(* Logix 5000 AddOnInstructionDefinition export Banner_RSio_ISD_Device_Information_v1; software revision 33.00 *)

TYPE Banner_RSio_ISD_Data_v1 :   // Tag Data for a Banner ISD Device.
STRUCT
   Safety_Input_Fault : SINT;   // System detected a fault on the safety input. Power cycle required. 1 = True, 0 = False.
   Reserved : SINT;
   Sensor_not_Paired : SINT;   // Si-RF Only. High or Unique sensor that has not been taught (not taught 1, taught 0)
   ISD_Data_Error : SINT;   // 1 = corrupted data was received by the Safety Controller, 0 = data ok.
   Wrong_Actuator : SINT;   // Si-RF sensor detects an actuator with a "received code" that does not match the "expected code" (wrong 1, correct 0).
   Marginal_Range : SINT;   // Si-RF Only. Actuator detected but is staying at the extreme end of detection range (13 to 15 mm away from sensor). 1 = True, 0 = False.
   Actuator_Detected : SINT;   // Si-RF sensor detects an actuator. Note: It does not have to be the taught actuator.
   Output_Error : SINT;   // ISD device detects an output short to voltage or ground. This starts the "switch-off timer" counter. 1= Error detected, 0 = OK.
   Input_1 : SINT;   // ISD device input 1 is on (1) or off (0)
   Input_2 : SINT;   // ISD device input 2 is on (1) or off (0)
   Local_Reset_Expected : SINT;   // An ISD device with latching feature requires a reset. 1 = reset needed. ISD Connect is always 0.
   Operating_Voltage_Warning : SINT;   // Voltage to the ISD device is at limit of specificaitons. 1 = at limit, 0 = OK.
   Operating_Voltage_Error : SINT;   // Voltage to the ISD device is above/over 30 Vdc or below/less 19.2 Vdc limit of range.
   Output_1 : SINT;   // 1 = Output On, 0 = Output Off
   Output_2 : SINT;   // 1 = Output On, 0 = Output Off
   Power_Cycle_Required : SINT;   // 1 = ISD device detects a fault. Power cycled required.
   Fault_Tolerant_Outputs : SINT;   // 1 = ISD device includes 20 minute off delay/fault delay. Always 1 for ISD E-Stop and ISD Connect.
   Local_Reset_Unit : SINT;   // 1 = ISD device includes the latch feature, 0 = device has the auto reset feature. Always 0 for ISD Connect.
   Cascadable : SINT;   // 1 = ISD device includes the cascade feature. Always 1 for ISD E-Stop and ISD Connect.
   High_Coding_Level : SINT;   // Si-RF Only. 1 = Device is High or Unique model, 0 = Low model.
   Teach_ins_Remaining : INT;   // Si-RF Only. Number of teaches remaining for Si-RF devices with high or unique coding.
   Device_Id : INT;   // ISD Device Type 1 = Si-RF. 7 for ISD E-Stop, 9 for ISD Connect.
   Range_Warning_Count : INT;   // Si-RF sensor only. Count of number of range warnings received in the last 60 minutes.
   Output_Switch_Out_Time : INT;   // Delay counter for certain output errors. 0 = inactive, 1 to 20 = remaining minutes to device lockout state. Value = 31 means Timer is Off.
   Number_of_Voltage_Errors : INT;   // 0 to 60 = Number of voltage warnings received in the last 60 seconds.
   Internal_Temperature : REAL;   // Internal temperature of device in Celsius.
   Actuator_Distance : REAL;   // The distance the actuator is from the Si-RF. Value displayed as a percentage of the Si-RF range.
   Supply_Voltage : REAL;   // Actual input voltage detected by the ISD sensor.
   Expected_Company_Name : INT;   // Fixed value of 6.
   Received_Company_Name : INT;   // Si-RF Only. Value received from Sensor. Should match Expected Company Name.
   Expected_Code : INT;   // Si-RF sensor with high or unique coding displays the actuator code taught to the sensor.
   Received_Code : INT;   // Displays actuator code detected by the Si-RF sensor.
   Internal_Error_A : DINT;
   Internal_Error_B : DINT;
END_STRUCT
END_TYPE

TYPE Banner_RSio_ISD_Device_Info_v1 :
STRUCT
   Chain : SINT;   // Enter Chain that will be accessed.
   Device : SINT;   // Enter Device that will be accessed.
   AccessChainDevice : SINT[2];
   RawInfo : SINT[18];
   DeviceInfo : Banner_RSio_ISD_Data_v1;
END_STRUCT
END_TYPE

ADD_ON_INSTRUCTION Banner_RSio_ISD_Device_Information_v1   (* revision 1.0 *)
VAR_IN_OUT
   ISD_Device : Banner_RSio_ISD_Device_Info_v1; {required}
   MSG : MESSAGE; {required}
   Activate : BOOL; {required}
END_VAR
VAR_OUTPUT
   Busy : BOOL; {visible}
   Done : BOOL; {visible}
   Error : BOOL; {visible}
END_VAR
VAR
   Control : DINT; {access None}
   Timer : TIMER := (PRE := 6000); {access None}
   T_Voltage : DINT; {access None}
   T_Temp : DINT; {access None}
   T_Distance : DINT; {access None}
   Temp2 : DINT[31]; {access None}
   Temp1 : DINT[31]; {access None}
   Distance2 : DINT[13] := ([1] := 7, [2] := 8, [3] := 9, [4] := 10, [5] := 11, [6] := 12, [7] := 13, [8] := 14, [9] := 15, [10] := 16, [11] := 17, [12] := 18); {access None}
   Distance1 : DINT[13] := ([0] := 61, [1] := 62, [2] := 65, [3] := 77, [4] := 110, [5] := 133, [6] := 148, [7] := 158, [8] := 163, [9] := 169, [10] := 172, [11] := 176, [12] := 180); {access None}
   IndexD : DINT; {access None}
   IndexT : DINT; {access None}
   Shift_T : DINT; {access None}
END_VAR

ROUTINE Logic   (* ladder *)
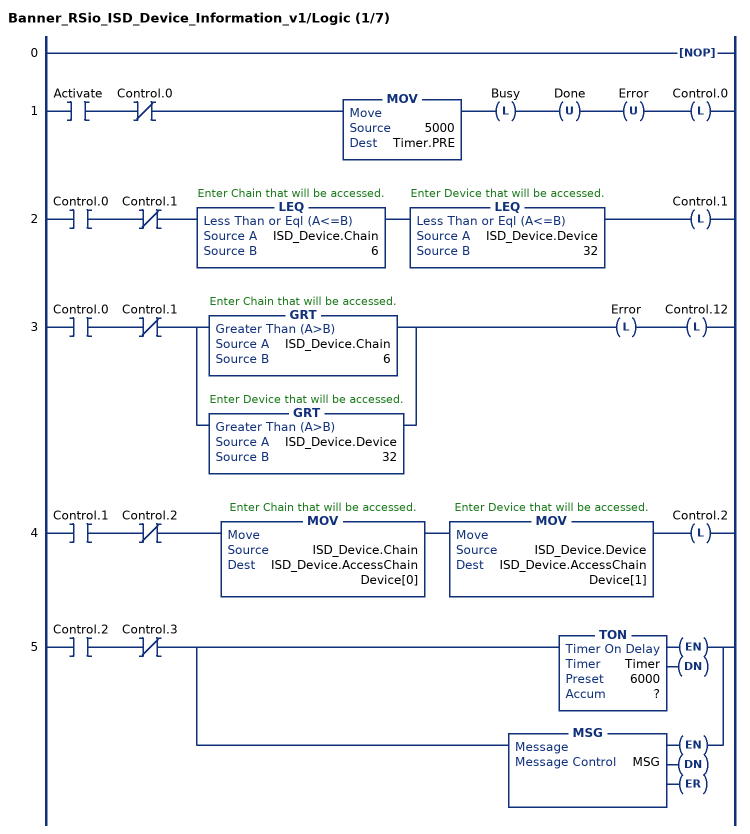
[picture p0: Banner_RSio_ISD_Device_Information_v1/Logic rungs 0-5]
   0: NOP();
   1: XIC(Activate)XIO(Control.0)MOV(5000,Timer.PRE)OTL(Busy)OTU(Done)OTU(Error)OTL(Control.0);
   2: XIC(Control.0)XIO(Control.1)LEQ(ISD_Device.Chain,6)LEQ(ISD_Device.Device,32)OTL(Control.1);
   3: XIC(Control.0)XIO(Control.1)[GRT(ISD_Device.Chain,6) ,GRT(ISD_Device.Device,32) ]OTL(Error)OTL(Control.12);
   4: XIC(Control.1)XIO(Control.2)MOV(ISD_Device.Chain,ISD_Device.AccessChainDevice[0])MOV(ISD_Device.Device,ISD_Device.AccessChainDevice[1])OTL(Control.2);
   5: XIC(Control.2)XIO(Control.3)[TON(Timer,?,?) ,MSG(MSG) ];
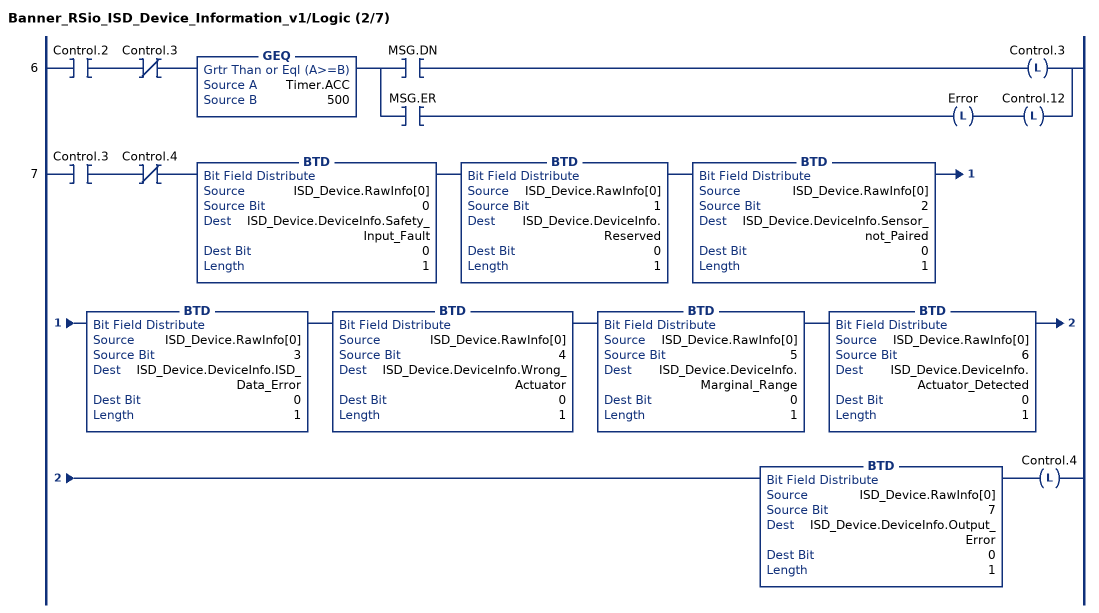
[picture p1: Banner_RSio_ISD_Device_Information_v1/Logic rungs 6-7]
   6: XIC(Control.2)XIO(Control.3)GEQ(Timer.ACC,500)[XIC(MSG.DN) OTL(Control.3) ,XIC(MSG.ER) OTL(Error) OTL(Control.12) ];
   7: XIC(Control.3)XIO(Control.4)BTD(ISD_Device.RawInfo[0],0,ISD_Device.DeviceInfo.Safety_Input_Fault,0,1)BTD(ISD_Device.RawInfo[0],1,ISD_Device.DeviceInfo.Reserved,0,1)BTD(ISD_Device.RawInfo[0],2,ISD_Device.DeviceInfo.Sensor_not_Paired,0,1)BTD(ISD_Device.RawInfo[0],3,ISD_Device.DeviceInfo.ISD_Data_Error,0,1)BTD(ISD_Device.RawInfo[0],4,ISD_Device.DeviceInfo.Wrong_Actuator,0,1)BTD(ISD_Device.RawInfo[0],5,ISD_Device.DeviceInfo.Marginal_Range,0,1)BTD(ISD_Device.RawInfo[0],6,ISD_Device.DeviceInfo.Actuator_Detected,0,1)BTD(ISD_Device.RawInfo[0],7,ISD_Device.DeviceInfo.Output_Error,0,1)OTL(Control.4);
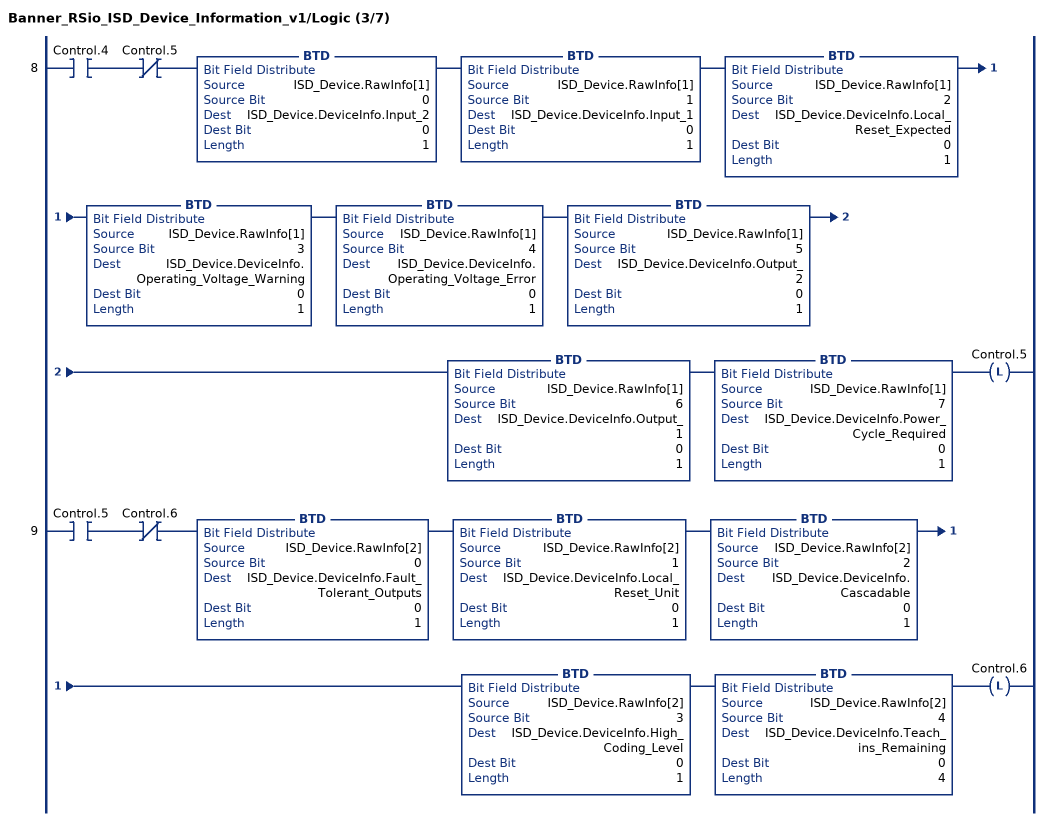
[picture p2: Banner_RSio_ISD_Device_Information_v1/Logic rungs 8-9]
   8: XIC(Control.4)XIO(Control.5)BTD(ISD_Device.RawInfo[1],0,ISD_Device.DeviceInfo.Input_2,0,1)BTD(ISD_Device.RawInfo[1],1,ISD_Device.DeviceInfo.Input_1,0,1)BTD(ISD_Device.RawInfo[1],2,ISD_Device.DeviceInfo.Local_Reset_Expected,0,1)BTD(ISD_Device.RawInfo[1],3,ISD_Device.DeviceInfo.Operating_Voltage_Warning,0,1)BTD(ISD_Device.RawInfo[1],4,ISD_Device.DeviceInfo.Operating_Voltage_Error,0,1)BTD(ISD_Device.RawInfo[1],5,ISD_Device.DeviceInfo.Output_2,0,1)BTD(ISD_Device.RawInfo[1],6,ISD_Device.DeviceInfo.Output_1,0,1)BTD(ISD_Device.RawInfo[1],7,ISD_Device.DeviceInfo.Power_Cycle_Required,0,1)OTL(Control.5);
   9: XIC(Control.5)XIO(Control.6)BTD(ISD_Device.RawInfo[2],0,ISD_Device.DeviceInfo.Fault_Tolerant_Outputs,0,1)BTD(ISD_Device.RawInfo[2],1,ISD_Device.DeviceInfo.Local_Reset_Unit,0,1)BTD(ISD_Device.RawInfo[2],2,ISD_Device.DeviceInfo.Cascadable,0,1)BTD(ISD_Device.RawInfo[2],3,ISD_Device.DeviceInfo.High_Coding_Level,0,1)BTD(ISD_Device.RawInfo[2],4,ISD_Device.DeviceInfo.Teach_ins_Remaining,0,4)OTL(Control.6);
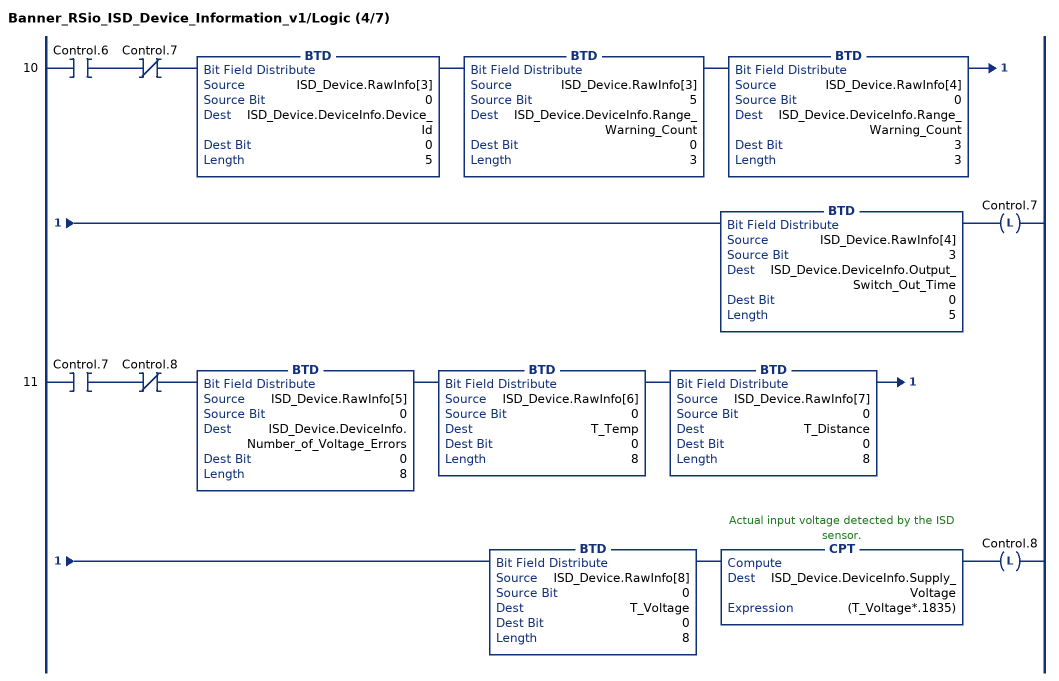
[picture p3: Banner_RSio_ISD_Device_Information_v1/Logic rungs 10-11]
   10: XIC(Control.6)XIO(Control.7)BTD(ISD_Device.RawInfo[3],0,ISD_Device.DeviceInfo.Device_Id,0,5)BTD(ISD_Device.RawInfo[3],5,ISD_Device.DeviceInfo.Range_Warning_Count,0,3)BTD(ISD_Device.RawInfo[4],0,ISD_Device.DeviceInfo.Range_Warning_Count,3,3)BTD(ISD_Device.RawInfo[4],3,ISD_Device.DeviceInfo.Output_Switch_Out_Time,0,5)OTL(Control.7);
   11: XIC(Control.7)XIO(Control.8)BTD(ISD_Device.RawInfo[5],0,ISD_Device.DeviceInfo.Number_of_Voltage_Errors,0,8)BTD(ISD_Device.RawInfo[6],0,T_Temp,0,8)BTD(ISD_Device.RawInfo[7],0,T_Distance,0,8)BTD(ISD_Device.RawInfo[8],0,T_Voltage,0,8)CPT(ISD_Device.DeviceInfo.Supply_Voltage,(T_Voltage*.1835))OTL(Control.8);
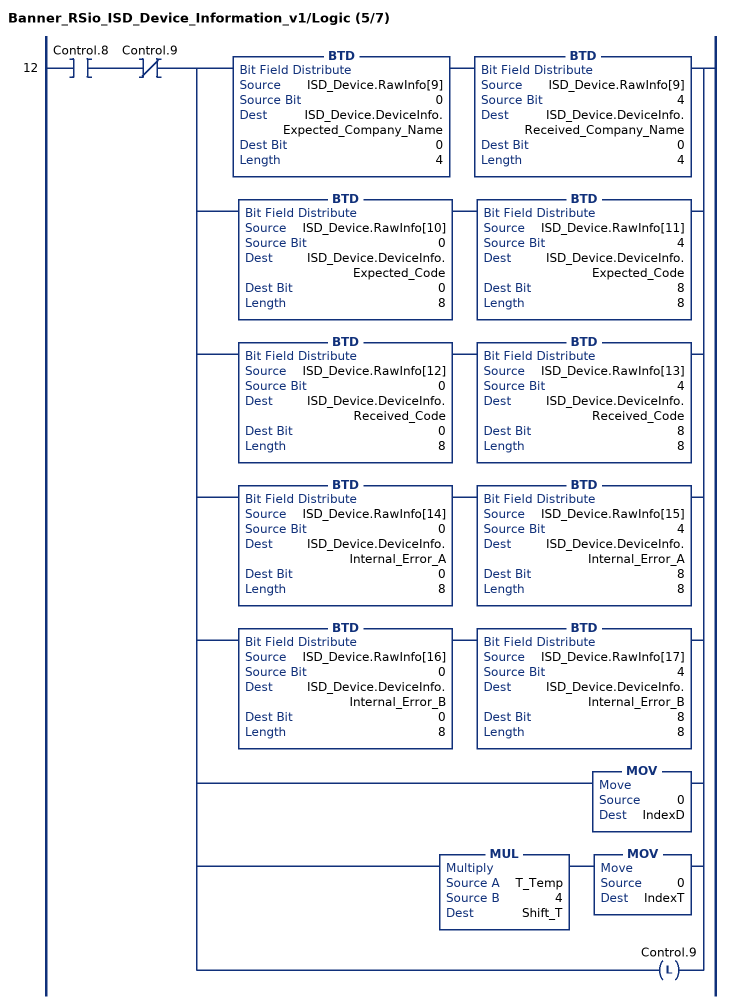
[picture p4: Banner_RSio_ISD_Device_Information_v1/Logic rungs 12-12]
   12: XIC(Control.8)XIO(Control.9)[BTD(ISD_Device.RawInfo[9],0,ISD_Device.DeviceInfo.Expected_Company_Name,0,4) BTD(ISD_Device.RawInfo[9],4,ISD_Device.DeviceInfo.Received_Company_Name,0,4) ,BTD(ISD_Device.RawInfo[10],0,ISD_Device.DeviceInfo.Expected_Code,0,8) BTD(ISD_Device.RawInfo[11],4,ISD_Device.DeviceInfo.Expected_Code,8,8) ,BTD(ISD_Device.RawInfo[12],0,ISD_Device.DeviceInfo.Received_Code,0,8) BTD(ISD_Device.RawInfo[13],4,ISD_Device.DeviceInfo.Received_Code,8,8) ,BTD(ISD_Device.RawInfo[14],0,ISD_Device.DeviceInfo.Internal_Error_A,0,8) BTD(ISD_Device.RawInfo[15],4,ISD_Device.DeviceInfo.Internal_Error_A,8,8) ,BTD(ISD_Device.RawInfo[16],0,ISD_Device.DeviceInfo.Internal_Error_B,0,8) BTD(ISD_Device.RawInfo[17],4,ISD_Device.DeviceInfo.Internal_Error_B,8,8) ,MOV(0,IndexD) ,MUL(T_Temp,4,Shift_T) MOV(0,IndexT) ,OTL(Control.9) ];
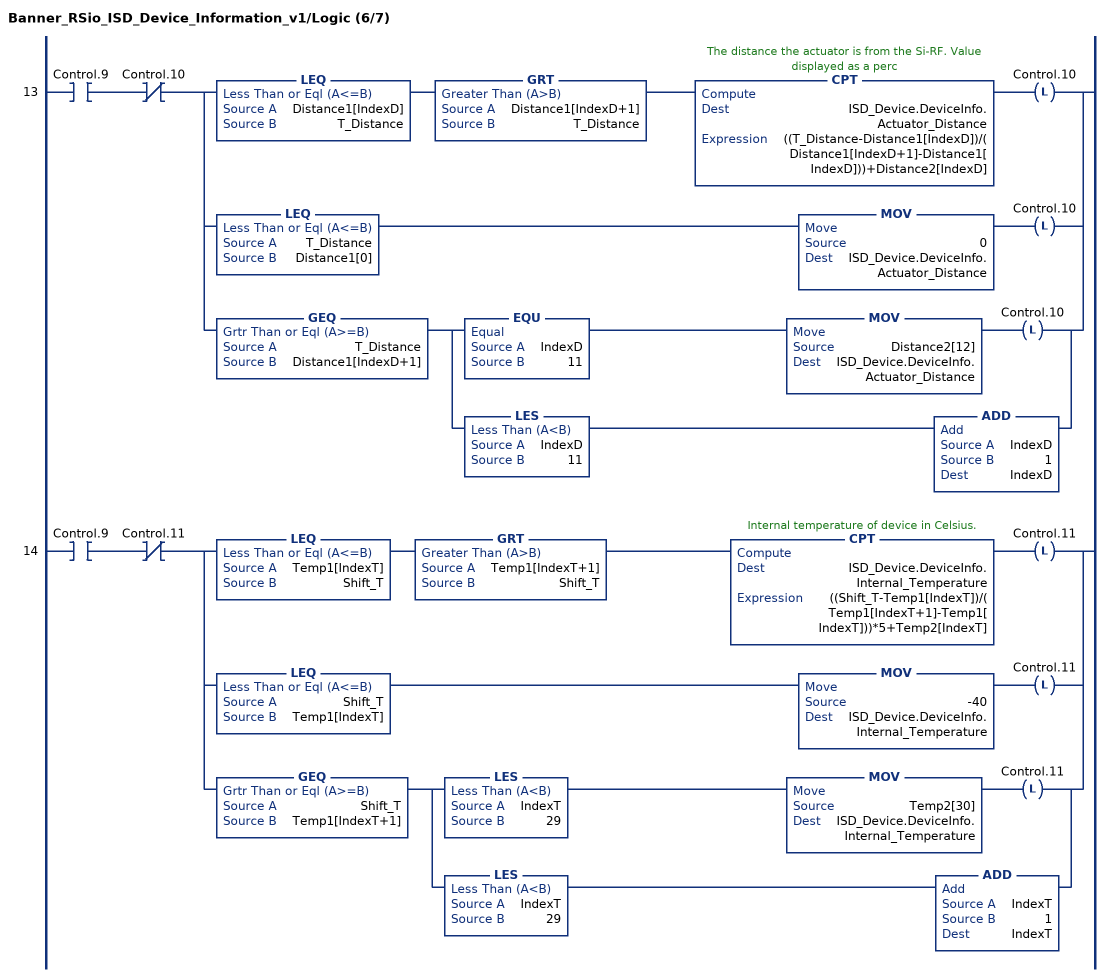
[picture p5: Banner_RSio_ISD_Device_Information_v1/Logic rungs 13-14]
   13: XIC(Control.9)XIO(Control.10)[LEQ(Distance1[IndexD],T_Distance) GRT(Distance1[IndexD+1],T_Distance) CPT(ISD_Device.DeviceInfo.Actuator_Distance,((T_Distance-Distance1[IndexD])/(Distance1[IndexD+1]-Distance1[IndexD]))+Distance2[IndexD]) OTL(Control.10) ,[LEQ(T_Distance,Distance1[0]) MOV(0,ISD_Device.DeviceInfo.Actuator_Distance) OTL(Control.10) ,GEQ(T_Distance,Distance1[IndexD+1]) [EQU(IndexD,11) MOV(Distance2[12],ISD_Device.DeviceInfo.Actuator_Distance) OTL(Control.10) ,LES(IndexD,11) ADD(IndexD,1,IndexD) ] ] ];
   14: XIC(Control.9)XIO(Control.11)[LEQ(Temp1[IndexT],Shift_T) GRT(Temp1[IndexT+1],Shift_T) CPT(ISD_Device.DeviceInfo.Internal_Temperature,((Shift_T-Temp1[IndexT])/(Temp1[IndexT+1]-Temp1[IndexT]))*5+Temp2[IndexT]) OTL(Control.11) ,[LEQ(Shift_T,Temp1[IndexT]) MOV(-40,ISD_Device.DeviceInfo.Internal_Temperature) OTL(Control.11) ,GEQ(Shift_T,Temp1[IndexT+1]) [LES(IndexT,29) MOV(Temp2[30],ISD_Device.DeviceInfo.Internal_Temperature) OTL(Control.11) ,LES(IndexT,29) ADD(IndexT,1,IndexT) ] ] ];
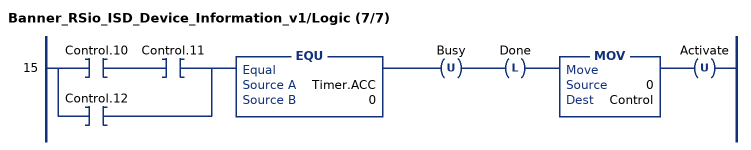
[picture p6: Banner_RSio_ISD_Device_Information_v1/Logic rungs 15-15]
   15: [XIC(Control.10) XIC(Control.11) ,XIC(Control.12) ]EQU(Timer.ACC,0)OTU(Busy)OTL(Done)MOV(0,Control)OTU(Activate);
END_ROUTINE
END_ADD_ON_INSTRUCTION
